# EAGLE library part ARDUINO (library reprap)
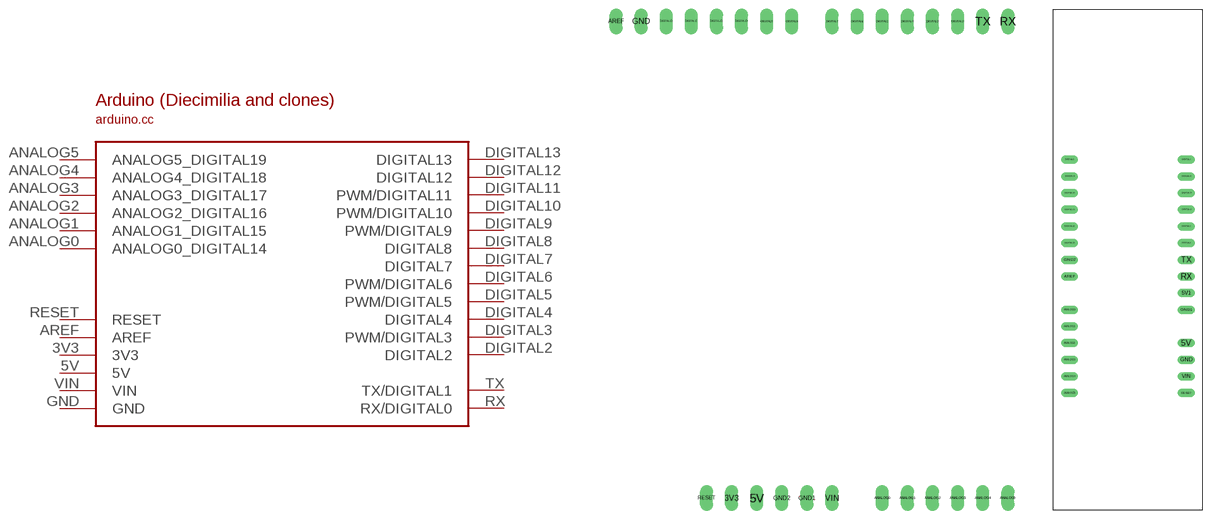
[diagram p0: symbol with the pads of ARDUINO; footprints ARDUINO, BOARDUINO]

Designator prefix -

## ARDUINODIECIMILIA  [ARDUINO]
3V3  3V3
5V  5V
ANALOG0  ANALOG0_DIGITAL14
ANALOG1  ANALOG1_DIGITAL15
ANALOG2  ANALOG2_DIGITAL16
ANALOG3  ANALOG3_DIGITAL17
ANALOG4  ANALOG4_DIGITAL18
ANALOG5  ANALOG5_DIGITAL19
AREF  AREF
DIGITAL2  DIGITAL2
DIGITAL3  PWM/DIGITAL3
DIGITAL4  DIGITAL4
DIGITAL5  PWM/DIGITAL5
DIGITAL6  PWM/DIGITAL6
DIGITAL7  DIGITAL7
DIGITAL8  DIGITAL8
DIGITAL9  PWM/DIGITAL9
DIGITAL10  PWM/DIGITAL10
DIGITAL11  PWM/DIGITAL11
DIGITAL12  DIGITAL12
DIGITAL13  DIGITAL13
GND  GND
RESET  RESET
RX  RX/DIGITAL0
TX  TX/DIGITAL1
VIN  VIN

## ARDUINO  [BOARDUINO]
5V  5V
ANALOG0  ANALOG0_DIGITAL14
ANALOG1  ANALOG1_DIGITAL15
ANALOG2  ANALOG2_DIGITAL16
ANALOG3  ANALOG3_DIGITAL17
ANALOG4  ANALOG4_DIGITAL18
ANALOG5  ANALOG5_DIGITAL19
AREF  AREF
DIGITAL2  DIGITAL2
DIGITAL3  PWM/DIGITAL3
DIGITAL4  DIGITAL4
DIGITAL5  PWM/DIGITAL5
DIGITAL6  PWM/DIGITAL6
DIGITAL7  DIGITAL7
DIGITAL8  DIGITAL8
DIGITAL9  PWM/DIGITAL9
DIGITAL10  PWM/DIGITAL10
DIGITAL11  PWM/DIGITAL11
DIGITAL12  DIGITAL12
DIGITAL13  DIGITAL13
GND  GND
GND1  3V3
RESET  RESET
RX  RX/DIGITAL0
TX  TX/DIGITAL1
VIN  VIN

## Footprint ARDUINO (pad centres in mm)
drill 0.8 long: 3V3 6.604,-45.72; 5V 9.144,-45.72; ANALOG0 21.844,-45.72; ANALOG1 24.384,-45.72; ANALOG2 26.924,-45.72; ANALOG3 29.464,-45.72; ANALOG4 32.004,-45.72; ANALOG5 34.544,-45.72; AREF -5.08,2.54; DIGITAL2 29.464,2.54; DIGITAL3 26.924,2.54; DIGITAL4 24.384,2.54; DIGITAL5 21.844,2.54; DIGITAL6 19.304,2.54; DIGITAL7 16.764,2.54; DIGITAL8 12.7,2.54; DIGITAL9 10.16,2.54; DIGITAL10 7.62,2.54; DIGITAL11 5.08,2.54; DIGITAL12 2.54,2.54; DIGITAL13 0,2.54; GND -2.54,2.54; GND1 14.224,-45.72; GND2 11.684,-45.72; RESET 4.064,-45.72; RX 34.544,2.54; TX 32.004,2.54; VIN 16.764,-45.72

## Footprint BOARDUINO (pad centres in mm)
drill 0.8 long: 5V 0,7.62; 5V1 0,15.24; ANALOG0 -17.78,12.7; ANALOG1 -17.78,10.16; ANALOG2 -17.78,7.62; ANALOG3 -17.78,5.08; ANALOG4 -17.78,2.54; ANALOG5 -17.78,0; AREF -17.78,17.78; DIGITAL2 0,22.86; DIGITAL3 0,25.4; DIGITAL4 0,27.94; DIGITAL5 0,30.48; DIGITAL6 0,33.02; DIGITAL7 0,35.56; DIGITAL8 -17.78,35.56; DIGITAL9 -17.78,33.02; DIGITAL10 -17.78,30.48; DIGITAL11 -17.78,27.94; DIGITAL12 -17.78,25.4; DIGITAL13 -17.78,22.86; GND 0,5.08; GND1 0,12.7; GND2 -17.78,20.32; RESET 0,0; RX 0,17.78; TX 0,20.32; VIN 0,2.54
